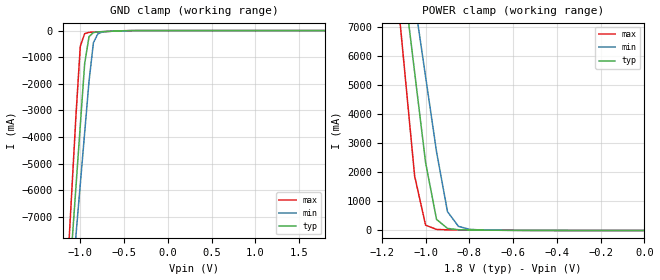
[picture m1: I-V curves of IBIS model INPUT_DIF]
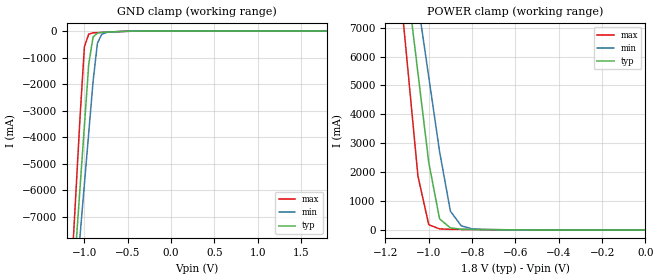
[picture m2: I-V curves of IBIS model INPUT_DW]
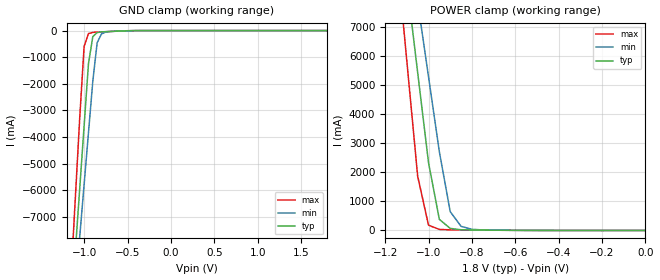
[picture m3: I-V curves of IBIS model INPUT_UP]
|   DIODES INCORPORATED
|   IBIS Model of PI6CB18401
|   Product Family: 6CB
|   TQFN 32-Pins (ZH) Package
[IBIS Ver] 4.0
[Comment char] |_char
[File Name] pi6cb18401_zh_reva.ibs
[File Rev] 1.0
[Source] File originated at Diodes Incorporated.
[Date] 12/19/18
[Disclaimer] (C) Copyright DIODES INCORPORATED
   All rights reserved
  Diodes Incorporated hereby grants the user of
  this IBIS model a non-exclusive, nontransferable license to
  use this IBIS model under the following terms.
  This IBIS model is provided on an "AS IS" basis and Diodes
  makes absolutely no warranty with respect to the information
  contained herein. DIODES DISCLAIMS AND CUSTOMER WAIVES ALL
  WARRANTIES, EXPRESSED OR IMPLIED, INCLUDING WARRANTIES OF
  MERCHANTABILITY OR FITNESS FOR A PARTICULAR PURPOSE. The
  entire risk as to quality and performance is with the customer.
  Accordingly, in no event shall the company be liable for any
  damages, whether in contract or tort, including any lost
  profits or other incidental, consequential, exemplary, or
  punitive damages arising out of the use or application of the
  IBIS model provided in this package. Further, Diodes reserves
  the right to make changes without notice to any product herein
  to improve reliability, function, or design. Diodes does not
  convey any license under patent rights or any other intellectual
  property rights, including those of third parties.
  The user is granted this license only to use the IBIS model
  and is not granted rights to sell, load, rent, lease or license
  the IBIS model in whole or in part, or in modified form to anyone
  other than user. User may modify the IBIS model to suit its specific
  application but rights to derivative works and such modifications
  shall belong to Diodes.
  Diodes is not obligated to provide maintenance or support
  for the licensed IBIS model.
  Contact Diodes at ATTN: APPLICATION ENGINEERING / IBIS MODELS
  1545 Barber Ln. Milpitas, CA 95035
[Component] PI6CB18401
[Manufacturer] Diodes Incorporated.
[Package]
| Variable   typ   min   max
R_pkg   0.03714ohm   0.02922ohm   0.04506ohm
L_pkg   0.78919nH   0.76828nH   0.81010nH
C_pkg   0.19084pF   0.17176pF   0.20992pF
[Pin]  signal_name   model_name   R_pin   L_pin   C_pin
1   BW_SEL_TRI   NC   0.04506   0.81010nH   0.20992pF
2   NC   NC   0.03978   0.79616nH   0.19720pF
3   NC   NC   0.03450   0.78222nH   0.18448pF
4   VDD_R   POWER   0.02922   0.76828nH   0.17176pF
5   IN+   INPUT_DIF   0.02922   0.76828nH   0.17176pF
6   IN-   INPUT_DIF   0.03450   0.78222nH   0.18448pF
7   GND_R   GND   0.03978   0.79616nH   0.19720pF
8   GND_DIG   GND   0.04506   0.81010nH   0.20992pF
9   VDD_DIG   POWER   0.04506   0.81010nH   0.20992pF
10   SCLK   INPUT_SCLK   0.03978   0.79616nH   0.19720pF
11   SDATA   IO   0.03450   0.78222nH   0.18448pF
12   OE0#   INPUT_DW   0.02922   0.76828nH   0.17176pF
13   Q0+   HCSL_OUT   0.02922   0.76828nH   0.17176pF
14   Q0-   HCSL_OUT   0.03450   0.78222nH   0.18448pF
15   GND   GND   0.03978   0.79616nH   0.19720pF
16   VDDO   POWER   0.04506   0.81010nH   0.20992pF
17   OE1#   INPUT_DW   0.04506   0.81010nH   0.20992pF
18   Q1+   HCSL_OUT   0.03978   0.79616nH   0.19720pF
19   Q1-   HCSL_OUT   0.03450   0.78222nH   0.18448pF
20   GNDA   GND   0.02922   0.76828nH   0.17176pF
21   VDDA   POWER   0.02922   0.76828nH   0.17176pF
22   Q2+   HCSL_OUT   0.03450   0.78222nH   0.18448pF
23   Q2-   HCSL_OUT   0.03978   0.79616nH   0.19720pF
24   OE2#   INPUT_DW   0.04506   0.81010nH   0.20992pF
25   VDDO   POWER   0.04506   0.81010nH   0.20992pF
26   GND   GND   0.03978   0.79616nH   0.19720pF
27   Q3+   HCSL_OUT   0.03450   0.78222nH   0.18448pF
28   Q3-   HCSL_OUT   0.02922   0.76828nH   0.17176pF
29   OE3#   INPUT_DW   0.02922   0.76828nH   0.17176pF
30   GND   GND   0.03450   0.78222nH   0.18448pF
31   PD#   INPUT_UP   0.03978   0.79616nH   0.19720pF
32   SS_SEL_TRI   INPUT_UP   0.04506   0.81010nH   0.20992pF
[Diff Pin] inv_pin vdiff  tdelay_typ tdelay_min tdelay_max
5   6   NA   NA   NA   NA
13   14   NA   NA   NA   NA
18   19   NA   NA   NA   NA
22   23   NA   NA   NA   NA
27   28   NA   NA   NA   NA
[Model selector] HCSL_OUT
HCSL_0P6_SLOW  Diff Output,Amplitude=0.6V,SMBUS=2v/ns,slow,slew_rate=0
HCSL_0P6_FAST  Diff Output,Amplitude=0.6V,SMBUS=3v/ns,fast,slew_rate=1
HCSL_0P7_SLOW  Diff Output,Amplitude=0.7V,SMBUS=2v/ns,slow,slew_rate=0
HCSL_0P7_FAST  Diff Output,Amplitude=0.7V,SMBUS=3v/ns,fast,slew_rate=1
HCSL_0P8_SLOW  Diff Output,Amplitude=0.8V,SMBUS=2v/ns,slow,slew_rate=0
HCSL_0P8_FAST  Diff Output,Amplitude=0.8V,SMBUS=3v/ns,fast,slew_rate=1
HCSL_0P9_SLOW  Diff Output,Amplitude=0.9V,SMBUS=2v/ns,slow,slew_rate=0
HCSL_0P9_FAST  Diff Output,Amplitude=0.9V,SMBUS=3v/ns,fast,slew_rate=1
| Models and submodels in the file (13): INPUT_DIF (Input), INPUT_DW (Input), INPUT_UP (Input), INPUT_SCLK (Input), IO (I/O_open_drain), HCSL_0P6_FAST (Output), HCSL_0P6_SLOW (Output), HCSL_0P7_FAST (Output), HCSL_0P7_SLOW (Output), HCSL_0P8_FAST (Output), HCSL_0P8_SLOW (Output), HCSL_0P9_FAST (Output), HCSL_0P9_SLOW (Output)
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|   Model INPUT_DIF
[Model] INPUT_DIF
Model_type Input
Vinl = 540.00mV
Vinh = 1.2600V
| variable   typ   min   max
C_comp   1.000pF   0.997pF   2.003pF
[Voltage Range]   1.8000V   1.7000V   1.9000V
[POWER Clamp Reference]   1.8000V   1.7000V   1.9000V
[GND Clamp Reference]   0.0000V   0.0000V   0.0000V
[Temperature Range]   25   85   -40
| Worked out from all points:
|   GND clamp passes 1 mA (typ) near -0.38 V on its own axis
|   POWER clamp passes 1 mA (typ) near -0.45 V on its own axis
[GND Clamp]
| Voltage   I(typ)   I(min)   I(max)
-1.8V     -40.8A     -36.77A    -47.86A
-1.15V    -10.55A    -11.59A    -9.184A
-1.1V     -8.222A    -9.649A    -6.209A
-1.05V    -5.896A    -7.712A    -3.234A
-1V       -3.569A    -5.775A    -591.1mA
-950mV    -1.243A    -3.838A    -113.6mA
-900mV    -226.2mA   -1.902A    -67.1mA
-850mV    -74.81mA   -458.6mA   -57.3mA
-800mV    -48.92mA   -124.4mA   -50.76mA
-750mV    -40.1mA    -53.68mA   -43.2mA
-350mV    -370.5uA   -927.1uA   -74.54uA
1.8V      1.6nA      277.6nA    24.82pA
[POWER Clamp]
| Voltage   I(typ)   I(min)   I(max)
-1.8V     52A        46.64A     61.4A
-1.15V    11.65A     13.04A     9.805A
-1.1V     8.543A     10.46A     5.838A
-1.05V    5.441A     7.877A     1.87A
-1V       2.338A     5.294A     182.4mA
-950mV    382.2mA    2.711A     36.45mA
-900mV    71.6mA     649.3mA    21.67mA
-850mV    24.87mA    142.8mA    18.04mA
-800mV    16.12mA    40.15mA    15.3mA
-750mV    12.63mA    17.74mA    12.39mA
0V        1.6nA      43.78nA    28.91pA
|   Model INPUT_DW
[Model] INPUT_DW
Model_type Input
Vinl = 540.00mV
Vinh = 1.2600V
| variable   typ   min   max
C_comp   1.000pF   0.997pF   2.003pF
[Voltage Range]   1.8000V   1.7000V   1.9000V
[POWER Clamp Reference]   1.8000V   1.7000V   1.9000V
[GND Clamp Reference]   0.0000V   0.0000V   0.0000V
[Temperature Range]   25   85   -40
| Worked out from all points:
|   GND clamp passes 1 mA (typ) near -0.38 V on its own axis
|   POWER clamp passes 1 mA (typ) near -0.45 V on its own axis
[GND Clamp]
| Voltage   I(typ)   I(min)   I(max)
-1.8V     -40.8A     -36.77A    -47.86A
-1.15V    -10.55A    -11.59A    -9.184A
-1.1V     -8.222A    -9.649A    -6.209A
-1.05V    -5.896A    -7.712A    -3.234A
-1V       -3.569A    -5.775A    -591.1mA
-950mV    -1.243A    -3.838A    -113.6mA
-900mV    -226.2mA   -1.902A    -67.1mA
-850mV    -74.82mA   -458.6mA   -57.31mA
-800mV    -48.93mA   -124.4mA   -50.76mA
-750mV    -40.11mA   -53.69mA   -43.2mA
-350mV    -373.5uA   -930.2uA   -77.22uA
1.8V      14.98uA    16.02uA    13.77uA
[POWER Clamp]
| Voltage   I(typ)   I(min)   I(max)
-1.8V     52A        46.64A     61.4A
-1.15V    11.65A     13.04A     9.805A
-1.1V     8.543A     10.46A     5.838A
-1.05V    5.441A     7.877A     1.87A
-1V       2.338A     5.294A     182.5mA
-950mV    382.2mA    2.711A     36.48mA
-900mV    71.62mA    649.3mA    21.69mA
-850mV    24.89mA    142.9mA    18.06mA
-800mV    16.15mA    40.17mA    15.32mA
-750mV    12.65mA    17.76mA    12.41mA
0V        14.98uA    14.91uA    14.54uA
|   Model INPUT_UP
[Model] INPUT_UP
Model_type Input
Vinl = 540.00mV
Vinh = 1.2600V
| variable   typ   min   max
C_comp   1.000pF   0.997pF   2.003pF
[Voltage Range]   1.8000V   1.7000V   1.9000V
[POWER Clamp Reference]   1.8000V   1.7000V   1.9000V
[GND Clamp Reference]   0.0000V   0.0000V   0.0000V
[Temperature Range]   25   85   -40
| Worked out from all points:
|   GND clamp passes 1 mA (typ) near -0.38 V on its own axis
|   POWER clamp passes 1 mA (typ) near -0.45 V on its own axis
[GND Clamp]
| Voltage   I(typ)   I(min)   I(max)
-1.8V     -40.8A     -36.77A    -47.86A
-1.15V    -10.55A    -11.59A    -9.184A
-1.1V     -8.222A    -9.649A    -6.209A
-1.05V    -5.896A    -7.712A    -3.234A
-1V       -3.569A    -5.775A    -591.1mA
-950mV    -1.243A    -3.838A    -113.7mA
-900mV    -226.2mA   -1.902A    -67.12mA
-850mV    -74.83mA   -458.6mA   -57.32mA
-800mV    -48.94mA   -124.4mA   -50.78mA
-750mV    -40.12mA   -53.71mA   -43.22mA
-350mV    -388.4uA   -945.1uA   -91.75uA
1.8V      1.6nA      1.152uA    -765nA
[POWER Clamp]
| Voltage   I(typ)   I(min)   I(max)
-1.8V     52A        46.64A     61.4A
-1.15V    11.65A     13.04A     9.805A
-1.1V     8.543A     10.46A     5.838A
-1.05V    5.441A     7.877A     1.87A
-1V       2.338A     5.294A     182.4mA
-950mV    382.2mA    2.711A     36.46mA
-900mV    71.6mA     649.3mA    21.68mA
-850mV    24.88mA    142.8mA    18.05mA
-800mV    16.13mA    40.15mA    15.31mA
-750mV    12.64mA    17.75mA    12.39mA
0V        1.6nA      43.78nA    28.91pA
